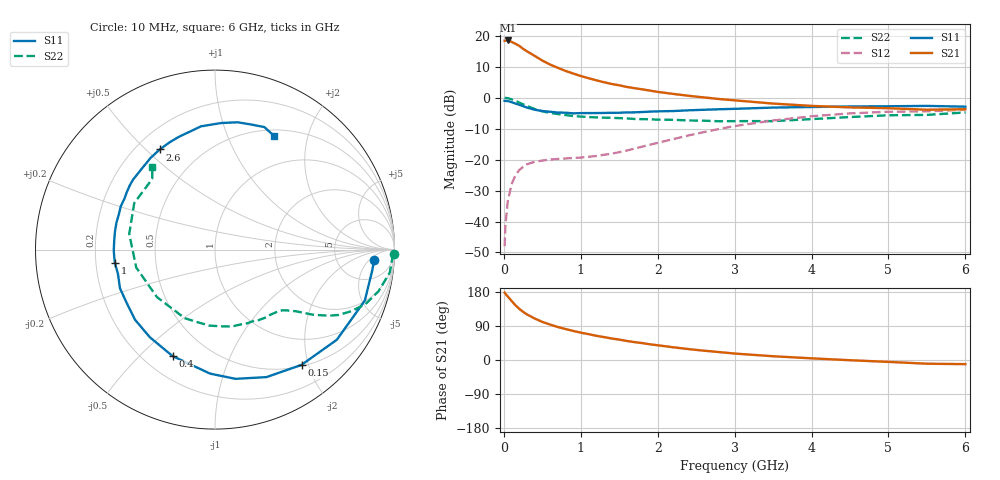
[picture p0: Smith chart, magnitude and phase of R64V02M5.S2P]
! SIEMENS Small Signal Semiconductors
! BFR193
! Si NPN RF Bipolar Junction Transistor in SOT23
! VCE = 4 V  IC = 2.5 mA
! Common Emitter S-Parameters:  May  1996
# GHz  S  MA  R  50
!  f  S11  S21  S12  S22
! GHz  MAG  ANG  MAG  ANG  MAG  ANG  MAG  ANG
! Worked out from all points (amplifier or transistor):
!   36 points, 10 MHz to 6 GHz, reference 50 ohm
!   highest |S21| = 18.5 dB at 50 MHz (marker M1)
!   |S21| within 3 dB of that: start of sweep to 269.1 MHz
!   unconditionally stable (mu >= 1): 1.103 GHz to 2.019 GHz
!   at 250 MHz: K = 0.27, MSG = 19.1 dB, |S12| = -22.3 dB
!   at 1.4 GHz: K = 1.10, MAG = 9.3 dB, |S12| = -18.1 dB
!   at 6 GHz: K = 0.99, MSG = 0.1 dB, |S12| = -3.9 dB
!   S11 on the Smith chart (normalised r, x): 10 MHz: 13, -7; 150 MHz: 0.52, -1.89; 400 MHz: 0.31, -0.63; 1 GHz: 0.28, -0.06; 2.6 GHz: 0.29, +0.55; 6 GHz: 0.57, +1.49
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0.01  0.8881 -3.7  8.305 177.8  0.004 89.3  0.9967 -1.5
0.02  0.8839 -7.5  8.317 174.9  0.0083 84.8  0.9889 -2.9
0.05  0.8817 -18.8  8.381 167.6  0.0208 80.5  0.982 -7.5
0.1  0.8445 -36.5  7.948 156.0  0.0398 71.2  0.9402 -14.3
0.15  0.803 -53.1  7.421 144.4  0.0557 62.6  0.8916 -19.9
0.2  0.7662 -68.0  6.864 135.2  0.0676 55.8  0.8324 -24.4
0.25  0.729 -81.0  6.148 127.2  0.0764 50.7  0.7781 -27.9
0.3  0.6914 -92.3  5.602 120.4  0.0839 46.9  0.7343 -30.1
0.4  0.6386 -111.7  4.733 109.6  0.092 41.2  0.656 -33.6
0.5  0.6085 -126.6  3.969 100.6  0.0964 38.1  0.6 -35.8
0.6  0.5927 -138.8  3.432 93.6  0.1001 36.9  0.5684 -37.2
0.7  0.5743 -149.3  3.037 87.2  0.1023 36.4  0.5438 -38.8
0.8  0.5716 -157.8  2.707 81.8  0.1042 36.8  0.5235 -40.3
1  0.563 -172.6  2.236 72.2  0.1078 41.3  0.4948 -43.8
1.1  0.5641 -179.2  2.061 68.2  0.111 43.6  0.4868 -46.0
1.6  0.5778 155.3  1.488 50.2  0.1401 56.0  0.462 -58.3
2.2  0.6076 132.3  1.149 33.6  0.2138 62.0  0.4386 -77.8
2.6  0.6373 118.9  1.009 24.6  0.2779 59.8  0.4245 -94.3
3.5  0.6912 96.5  0.802 9.9  0.428 45.5  0.418 -140.8
4.5  0.7206 79.9  0.696 -0.6  0.557 25.6  0.4858 169.6
5.5  0.736 68.1  0.638 -9.8  0.6011 6.6  0.5268 131.6
6  0.7145 62.7  0.651 -10.9  0.6356 1.4  0.5769 127.3
